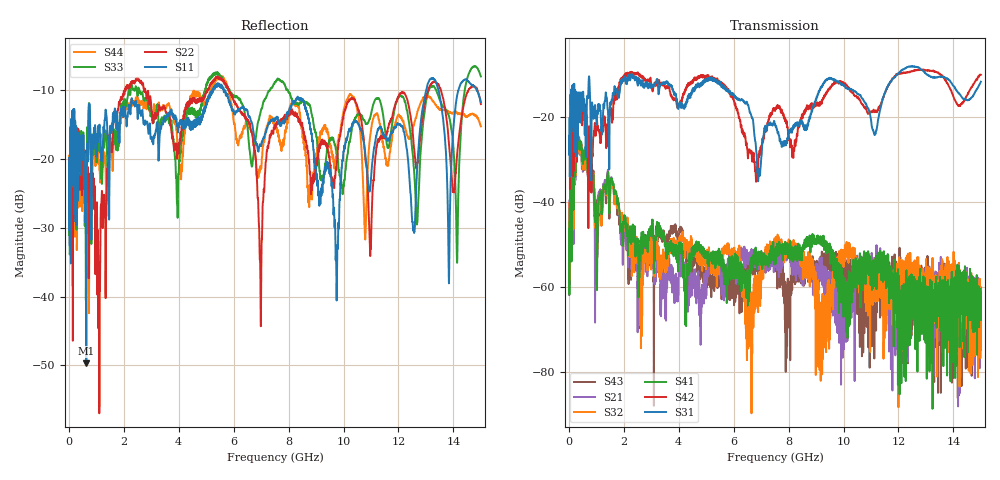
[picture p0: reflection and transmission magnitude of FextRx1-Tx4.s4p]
! FILE: N:\QM 2007\Prüfprotokolle\Highspeed\Konfektionierte Ltg\L45593-D106\D30\8216\0002\Fext\FextRx1-Tx4.s4p
# MHz S DB R 50.00
! FREQ  S11  S12  S13  S14
!  S21  S22  S23  S24
!  S31  S32  S33  S34
!  S41  S42  S43  S44
!  DB  ANG  DB  ANG  DB  ANG  DB  ANG
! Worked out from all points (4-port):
!   2999 points, 10 MHz to 15 GHz, reference 50 ohm
!   strongest paths, dB at 10 MHz, 3.755 GHz, 7.505 GHz, 11.26 GHz, 15 GHz:
!     S31: -25.5, -12.8, -21.7, -20.7, -11.7
!     S42: -24.7, -15.2, -18.6, -18.4, -10.1
!     S41: -52.4, -51.4, -51.9, -55.4, -67.8
!     S32: -45.3, -51.3, -49.6, -55.3, -74.8
!     S21: -45.4, -60.7, -53.1, -54.3, -68.9
!     S43: -40.3, -46.8, -54.9, -62.8, -70.3
!   lowest |S11| = -49.7 dB at 635 MHz (marker M1), VSWR 1.01, Z = 50.3 + j0.119 ohm
!   |S11| at or under -10 dB: start of sweep to 5.222 GHz; 5.665 GHz to 13.01 GHz (7.347 GHz wide, 78.7 % of centre); 13.46 GHz to 14.18 GHz (720.4 MHz wide, 5.21 % of centre)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
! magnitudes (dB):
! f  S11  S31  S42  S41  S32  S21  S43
! 10 MHz  -19.8  -25.5  -24.7  -52.4  -45.3  -45.4  -40.3
! 635 MHz  -49.7  -29.3  -23.9  -26.4  -27.9  -28.0  -26.8
! 2.625 GHz  -13.8  -12.6  -10.5  -48.6  -74.5  -55.3  -51.2
! 6.975 GHz  -18.1  -32.1  -27.5  -53.5  -56.6  -53.7  -56.4
! 8.07 GHz  -12.5  -23.1  -25.5  -52.3  -51.3  -53.5  -59.1
! 14.12 GHz  -11.0  -13.8  -16.9  -63.3  -59.1  -70.6  -61.6
! 15 GHz  -11.7  -11.7  -10.1  -67.8  -74.8  -68.9  -70.3
